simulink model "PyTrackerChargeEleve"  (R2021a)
settings: Solver=ode45  StartTime=0.0  StopTime=25000  RelTol=1e-3  EnableMultiTasking=on
libraries: fl_lib x4, nesl_utility x3, ee_lib x2

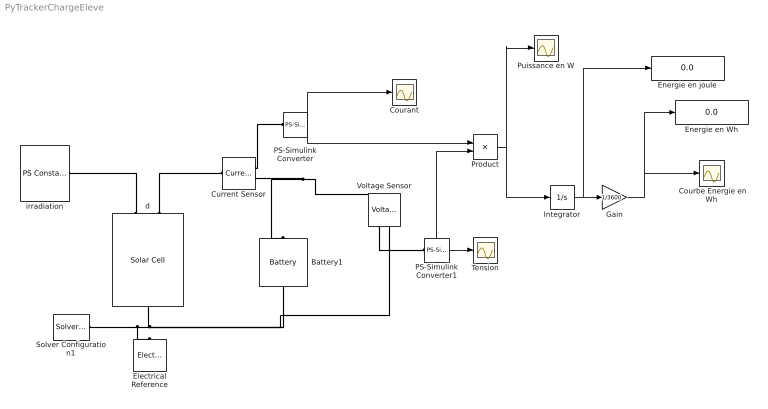
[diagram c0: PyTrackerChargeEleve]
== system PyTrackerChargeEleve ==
  " Courbe Energie en Wh" : Scope
  Battery1 : ee_lib/Sources/Battery  Vnom=13 V  prm_dir=1  R1_dis=2 Ohm  R1_ch=2 Ohm  R1=0.1 Ohm  prm_AH=2  AH=4 hr*A  V1=11.5 V  AH1=1 hr*A  prm_R2=2  R2=inf Ohm  prm_dyn=1  Rp1=0.005 Ohm  tau1=30 s  Rp2=0.005 Ohm  tau2=30 s  Rp3=0.005 Ohm  tau3=30 s  Rp4=0.005 Ohm  tau4=30 s  Rp5=0.005 Ohm  tau5=30 s  prm_fade=1  N_fade=100  AH_fade=45 hr*A  R1_fade=2.02 Ohm  R1_ch_fade=2.02 Ohm  V1_fade=10.35 V  prm_age=1  prm_age_OCV=1  OCV_age=0.9  SOC_age=60  Tmeas_age=298.15 K  delta_time_age_vec=[0] d  temperature_age_vec=[273] K  OCV_scaling_age=2.2134e6  OCV_offset_age=1.632e6  temp_exp_age=0.515833569 V  t_exp_age=0.75  i_specify=off  i_priority=None  i=0 A  i_nominal_specify=off  i_nominal_unit=A  i_nominal_value=1  v_specify=off  v_priority=None  v=0 V  v_nominal_specify=off  v_nominal_unit=V  v_nominal_value=1  charge_specify=on  charge_priority=High  charge=1 hr*A  charge_nominal_specify=off  charge_nominal_unit=hr*A  charge_nominal_value=1  num_cycles_specify=off  num_cycles_priority=High  num_cycles=0  num_cycles_nominal_specify=off  num_cycles_nominal_unit=1  num_cycles_nominal_value=1  thermal_mass=30000 J/K  Tmeas=298.15 K  Vnom_T2=12 V  R1_T2=2.2 Ohm  R1_T2_dis=2.2 Ohm  R1_T2_ch=2.2 Ohm  V1_T2=11.4 V  R2_T2=2200 Ohm  Rp1_T2=0.005 Ohm  tau1_T2=30 s  Rp2_T2=0.005 Ohm  tau2_T2=30 s  Rp3_T2=0.005 Ohm  tau3_T2=30 s  Rp4_T2=0.005 Ohm  tau4_T2=30 s  Rp5_T2=0.005 Ohm  tau5_T2=30 s  Tmeas2=273.15 K  temperature_specify=off  temperature_priority=High  temperature=298.15 K  temperature_nominal_specify=off  temperature_nominal_unit=K  temperature_nominal_value=1
  Courant : Scope
  Current Sensor : fl_lib/Electrical/Electrical Sensors/Current Sensor
  Electrical Reference : fl_lib/Electrical/Electrical Elements/Electrical Reference
  Energie en Wh : Display
  Energie en joule : Display
  Gain : Gain  Gain=1/3600
  Integrator : Integrator
  PS-Simulink Converter : nesl_utility/PS-Simulink Converter  PhysicalDomain=network_engine_domain  SubClassName=ps_output  LeftPortType=input  RightPortType=output  PseudoPeriodic=off  Frequencies=[]  Unit=A  AffineConversion=off
  PS-Simulink Converter1 : nesl_utility/PS-Simulink Converter  PhysicalDomain=network_engine_domain  SubClassName=ps_output  LeftPortType=input  RightPortType=output  PseudoPeriodic=off  Frequencies=[]  Unit=V  AffineConversion=off
  Product : Product
  Puissance en W : Scope
  Solver Configuration1 : nesl_utility/Solver Configuration  PhysicalDomain=network_engine_domain  SubClassName=solver  LeftPortType=input  RightPortType=generic  Tones=[]  Harmonics=[]  SimulateNoise=off  Profile=off  UseLocalSampling=off  EnableSwitchedLinearOptims=on  FrequencyDomain=off  UseCCode=off  RelTol=0.001  AbsTol=1e-06  MinStep=1e-09  ToWorkspace=off  RevertToSquareIcSolve=off  NumHomotopyIterations=100  PhasorMode=off  PhasorModeNumHarmonics=1  DoDC=off  ResidualTolerance=1e-09  UseLocalSolver=off  LocalSolverChoice=NE_BACKWARD_EULER_ADVANCER  LocalSolverSampleTime=0.001  DoFixedCost=off  MaxNonlinIter=3  MaxModeIter=2  ComputeImpulses=off  ImpulseIterations=2  LinearAlgebra=Sparse  EquationFormulation=NE_TIME_EF  DelaysMemoryBudget=1024  AutomaticFiltering=on  FilteringTimeConstant=0.001  PartitionStorageMethod=AS_NEEDED  PartitionMemoryBudget=1024  PartitionMethod=FAST
  Tension : Scope
  Voltage Sensor : fl_lib/Electrical/Electrical Sensors/Voltage Sensor
  d : ee_lib/Sources/Solar Cell  prm=1  Isc=0.32 A  Voc=21.6 V  Is=1e-6 A  Is2=0 A  Iph=7.34 A  Ir0=900 W/m^2  ec=1.5  N2=2  Rs=0 Ohm  Rp=Inf Ohm  N_series=35  TIPH1=0 1/K  EG=1.11 eV  TXIS1=3  TXIS2=3  TRS1=0  TRP1=0  Tmeas=25 degC  TFIXED=25 degC  thermal_mass=100 J/K  initial_temperature=25 degC
  irradiation : fl_lib/Physical Signals/Sources/PS Constant  constant=1000
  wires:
  PS-Simulink Converter/1 -> Product/1, Courant/1
  PS-Simulink Converter1/1 -> Product/2, Tension/1
  Product/1 -> Integrator/1, Puissance en W/1
  Integrator/1 -> Energie en joule/1, Gain/1
  Gain/1 -> Energie en Wh/1, " Courbe Energie en Wh"/1
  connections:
  Solver Configuration1/RConn1 -- Voltage Sensor/RConn2 -- Battery1/RConn1 -- Electrical Reference/LConn1 -- d/RConn1
  d/LConn1 -- irradiation/RConn1
  Current Sensor/RConn1 -- PS-Simulink Converter/LConn1
  d/LConn2 -- Current Sensor/LConn1
  Current Sensor/RConn2 -- Voltage Sensor/LConn1 -- Battery1/LConn1
  Voltage Sensor/RConn1 -- PS-Simulink Converter1/LConn1
